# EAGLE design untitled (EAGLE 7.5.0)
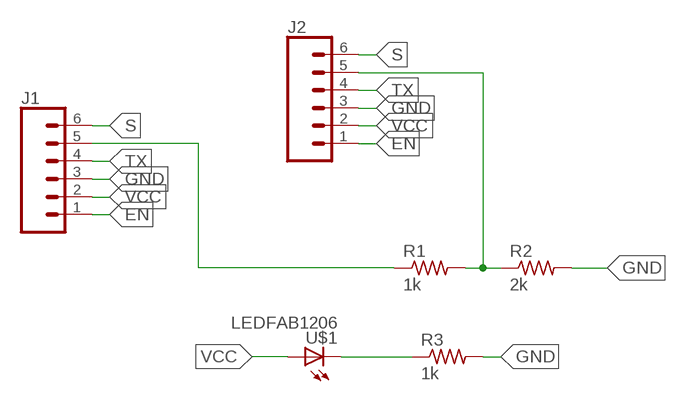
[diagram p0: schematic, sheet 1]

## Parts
J1  CONN_06SILK_FEMALE_PTH  [1X06]
J2  CONN_06SILK_FEMALE_PTH  [1X06]
R1  1k  RES-US1206FAB  [R1206FAB]
R2  2k  RES-US1206FAB  [R1206FAB]
R3  1k  RES-US1206FAB  [R1206FAB]
U$1  LEDFAB1206  [LED1206FAB]

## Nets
EN: J1.1 J2.1
GND: J1.3 J2.3 R2.2 R3.2
N$1: J2.5 R1.2 R2.1
N$3: J1.5 R1.1
N$4: R3.1 U$1.2(C)
S: J1.6 J2.6
TX: J1.4 J2.4
VCC: J1.2 J2.2 U$1.1(A)

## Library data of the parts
J1 J2 = SparkFun-Connectors:CONN_06: Multi connection point. Often used as Generic Header-pin footprint for 0.1 inch spaced/style header connections On any of the 0.1 inch spaced packages, you can populate with these: Break Away Headers - Straight (PRT-00116) Break Away Male Headers - Right Angle (PRT-00553) Female Headers (PRT-00115)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; PROD_ID: CONN-08437
R1-R3 = fab:RES-US: Resistor (US Symbol)
U$1 = fab:LED: LED

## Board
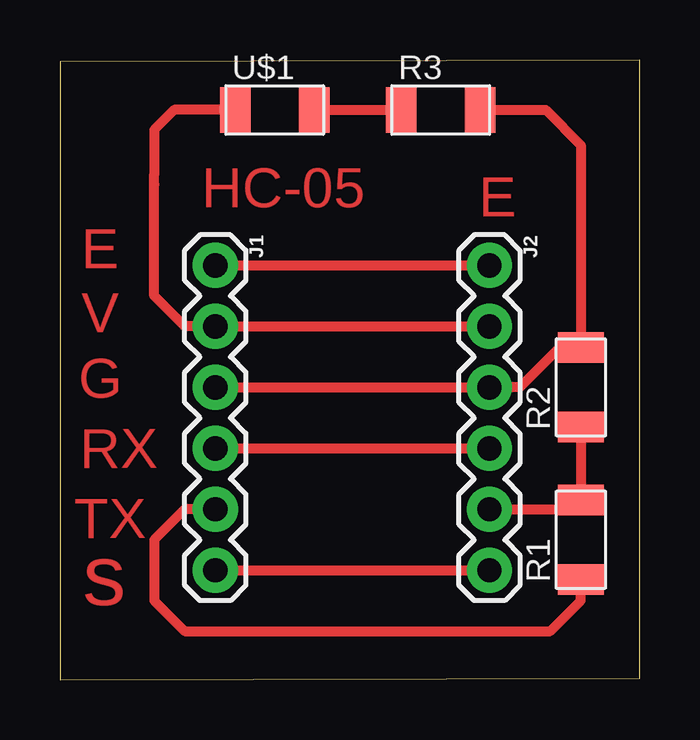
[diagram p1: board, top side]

Size 24.17 x 25.83 mm. Coordinates in mm from the lower left corner, seen from the top.
Outline: 0,0 24.17,0.06 24.17,25.83 0,25.77 0,0
Copper layers (1*16): Top 0.035mm / dielectric 1.5mm / Bottom 0.035mm
Design rules "default": minimum track width 10mil, minimum drill 24mil, track to track 8mil, track to pad 8mil, pad to pad 8mil, via to via 8mil, smd to smd 8mil, copper to edge 40mil, drill to drill 8mil, minimum pad ring 10mil, minimum via ring 8mil, stop-mask expansion 4mil, vias tented up to drill 0mil, thermal gap 10mil

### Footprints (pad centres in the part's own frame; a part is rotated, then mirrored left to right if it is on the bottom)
1X06 = drill 1.016 pad 1.88: 1 0,0; 2 2.54,0; 3 5.08,0; 4 7.62,0; 5 10.16,0; 6 12.7,0
R1206FAB = smd 1.27 x 1.905: 1 -1.651,0; 2 1.651,0
LED1206FAB = smd 1.27 x 1.905: 1 -1.651,0; 2 1.651,0

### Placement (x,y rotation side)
J1  6.48,17.27 270 top
J2  17.91,17.27 270 top
R1  21.72,5.84 90 top
R2  21.72,12.19 90 top
R3  15.88,23.75 0 top
U$1  8.95,23.75 0 top

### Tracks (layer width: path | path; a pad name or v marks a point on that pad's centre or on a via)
EN
  Top 0.406: J1.1 J2.1
GND
  Top 0.406: J1.3 J2.3 19.18,12.19 20.83,13.84 R2.2 21.72,22.29 20.26,23.75 R3.2
N$1
  Top 0.406: R2.1 R1.2 21.34,7.11 J2.5
N$3
  Top 0.406: J1.5 5.21,7.11 3.94,5.84 3.94,3.3 5.21,2.03 20.45,2.03 21.72,3.3 R1.1
N$4
  Top 0.406: U$1.2 R3.1
S
  Top 0.406: J1.6 J2.6
TX
  Top 0.406: J1.4 J2.4
VCC
  Top 0.406: J2.2 J1.2 5.21,14.73 3.94,16 3.94,20.64 3.94,21.08 3.94,22.92 4.76,23.75 U$1.1

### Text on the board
Top: HC-05 | E | E | V | G | RX | TX | s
